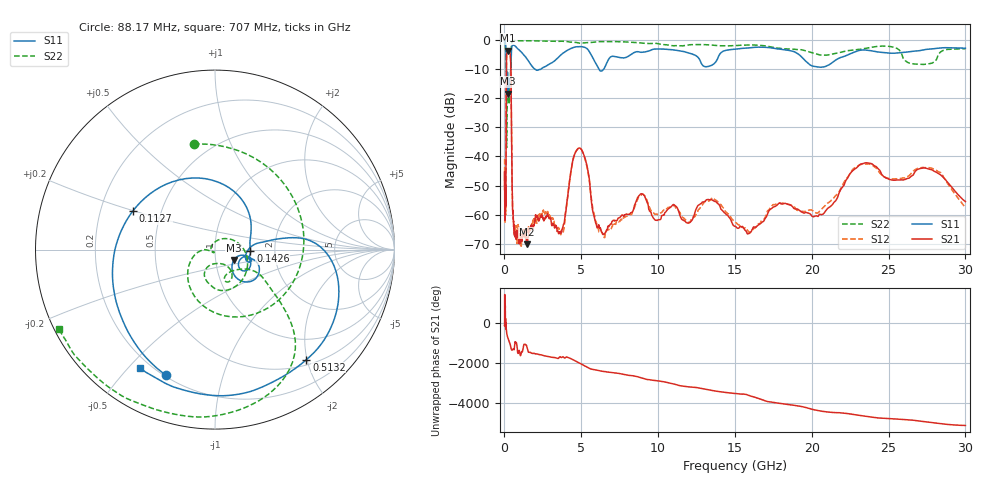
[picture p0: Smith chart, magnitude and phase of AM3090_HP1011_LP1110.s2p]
! Date/Time: Thu, Feb 28, 2019 2:06 PM
! Network Analyzer: Agilent Technologies E8364B Rev: A.07.50.67
! Sweep from 0.010 to 30.000 GHz, 1601 Points, Sweep Type: LOG
! Power Supply: 5.023 V, 0.002 A
# Hz S DB R 50
!freq MagS11 AngS11 MagS21 AngS21 MagS12 AngS12 MagS22 AngS22
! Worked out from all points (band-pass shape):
!   1601 points, 10 MHz to 30 GHz, reference 50 ohm
!   highest |S21| = -3.64 dB at 242.3 MHz (marker M1); lowest = -70.2 dB at 1.453 GHz (marker M2)
!   |S21| within 3 dB of the highest: 133.3 MHz to 399.8 MHz (266.5 MHz wide, 100 % of centre)
!   lowest |S11| = -18.4 dB at 243.5 MHz (marker M3), VSWR 1.27, Z = 61.3 - j7.21 ohm
!   |S11| at or under -10 dB: 124.7 MHz to 415.7 MHz (291 MHz wide, 108 % of centre); 1.972 GHz to 2.385 GHz (413 MHz wide, 19 % of centre); 6.145 GHz to 6.464 GHz (319.1 MHz wide, 5.06 % of centre)
!   |S22| runs from -37.0 to -0.2 dB; largest |S21 - S12| = 0.012
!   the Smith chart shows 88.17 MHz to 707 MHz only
!   S11 on the Smith chart (normalised r, x): 88.17 MHz: 0.21, -0.66; 112.7 MHz: 0.34, +0.20; 142.6 MHz: 1.49, -0.03; 513.2 MHz: 0.59, -1.99; 707 MHz: 0.16, -0.54
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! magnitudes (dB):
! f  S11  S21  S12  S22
! 10 MHz  -0.3  -51.4  -40.8  -0.6
! 38.04 MHz  -0.4  -58.3  -60.1  -1.6
! 88.17 MHz  -2.5  -56.0  -54.1  -4.5
! 112.7 MHz  -5.9  -26.0  -26.0  -6.7
! 142.6 MHz  -14.1  -5.2  -5.2  -34.8
! 144.7 MHz  -14.1  -5.0  -5.0  -34.1
! 181.3 MHz  -12.2  -3.9  -3.8  -14.8
! 242.3 MHz  -18.4  -3.6  -3.6  -14.0
! 243.5 MHz  -18.4  -3.6  -3.6  -14.0
! 405.7 MHz  -11.4  -7.3  -7.3  -8.9
! 513.2 MHz  -2.0  -55.2  -53.4  -0.5
! 550.5 MHz  -1.9  -59.3  -59.8  -0.4
! 707 MHz  -2.1  -65.9  -65.7  -0.2
! 1.453 GHz  -6.4  -70.2  -65.6  -0.3
! 2.084 GHz  -10.4  -60.5  -62.0  -0.3
! 3.742 GHz  -4.8  -65.0  -66.2  -0.4
! 4.854 GHz  -2.3  -37.1  -37.1  -1.1
! 6.265 GHz  -10.7  -65.1  -65.6  -0.6
! 7.926 GHz  -6.0  -59.8  -60.6  -0.7
! 16.05 GHz  -2.7  -65.9  -65.5  -1.7
! 23.48 GHz  -3.5  -42.2  -42.6  -2.9
! 30 GHz  -2.9  -55.5  -57.6  -3.0
